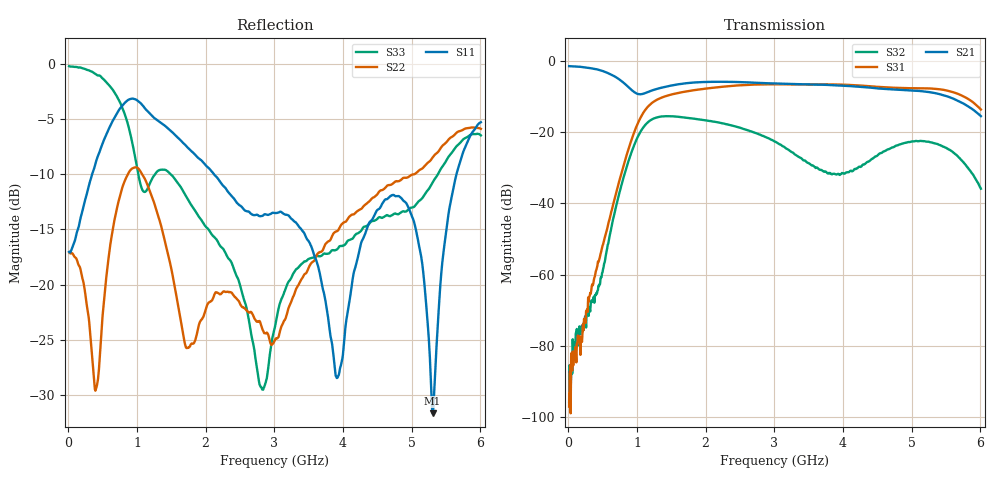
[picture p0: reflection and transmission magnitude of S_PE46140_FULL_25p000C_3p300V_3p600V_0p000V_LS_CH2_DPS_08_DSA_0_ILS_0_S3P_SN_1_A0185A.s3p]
! Device ID: PE46140_FULL
! File Path: z:\PE46140\MajorStates\25p000C\3p300\LS_CH2_DPS_08_DSA_0_ILS_0\PE46140_FULL_25p000C_3p300V_3p600V_0p000V_LS_CH2_DPS_08_DSA_0_ILS_0_S3P_SN_1_A0185A.s3p
! Serial: 1
! Lot: A0185A
! Temp: 25.000C
! VDD: 3.300
! VSS: 0.000
! Control_Hi: 3.600
! Control_Lo: 0.000
! Logic State: LS_CH2_DPS_08_DSA_0_ILS_0
! Port 1: RFIN
! Port 2: RFOUT1
! Port 3: RFOUT2
! ThroughPath:1-3
! IDD: 0.0003147101
! ISS: -1.246e-007
! Comment:
#  Hz  S  RI  R  50
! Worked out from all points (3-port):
!   801 points, 10 MHz to 6.01 GHz, reference 50 ohm
!   strongest paths, dB at 10 MHz, 1.51 GHz, 3.01 GHz, 4.51 GHz, 6.01 GHz:
!     S21: -1.5, -6.9, -6.4, -7.7, -15.5
!     S31: -97.0, -9.4, -6.6, -7.3, -13.7
!     S32: -95.7, -15.6, -22.7, -26.4, -35.9
!   lowest |S11| = -31.6 dB at 5.305 GHz (marker M1), VSWR 1.05, Z = 51.5 + j2.17 ohm
!   |S11| at or under -10 dB: start of sweep to 346.1 MHz; 2.119 GHz to 5.655 GHz (3.536 GHz wide, 91 % of centre)
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1e7  0.1402 -0.0109  0.842 -0.0245  -3.11e-05 3.34e-05
     0.8419 -0.0242  0.14 -0.00675  1.58e-05 1.55e-05
     -1.01e-05 -9.83e-06  1.38e-05 -8.72e-06  0.9729 -0.0266
4.075e8  -0.0696 -0.3583  0.3635 -0.6663  0.000303 -0.00112
         0.3648 -0.6704  -0.0311 -0.0145  -0.000562 3.68e-05
         0.000331 -0.00113  -0.000553 6.15e-05  0.5169 -0.7258
7.375e8  -0.5113 -0.3462  -0.1878 -0.5186  -0.00166 -0.02
         -0.1874 -0.5191  0.1397 0.1984  -0.0126 -0.00431
         -0.00172 -0.02  -0.0127 -0.00436  -0.1877 -0.6549
1.1425e9  -0.5829 0.1922  -0.2059 -0.2948  -0.1833 0.1181
          -0.2062 -0.2956  0.2292 -0.1731  0.0815 0.1052
          -0.1841 0.1181  0.0814 0.1053  -0.1694 -0.2075
1.8475e9  -0.1906 0.3363  -0.4832 0.1206  0.3783 -0.0913
          -0.4835 0.1205  0.0506 -0.0238  -0.15 -0.0311
          0.3789 -0.0914  -0.1503 -0.0312  -0.0922 0.1948
3.01e9  0.0105 0.2103  0.401 0.265  -0.465 -0.054
        0.4006 0.266  -0.056 -0.00182  0.0464 -0.0566
        -0.4655 -0.0545  0.0465 -0.0568  0.0203 0.0612
4.0675e9  -0.0237 -0.071  0.0104 -0.4443  0.1863 0.4218
          0.0112 -0.4445  0.1477 0.1313  0.0273 0.000723
          0.1865 0.4214  0.0273 0.000556  0.1366 0.0787
4.8475e9  -0.2447 0.0306  -0.3903 0.0197  0.3973 -0.1199
          -0.3909 0.0191  0.2977 0.0176  -0.0627 0.0265
          0.3976 -0.1199  -0.0625 0.0267  0.2115 -0.0201
5.305e9  0.0155 0.0211  -0.1485 0.3258  0.1531 -0.3784
         -0.1494 0.3259  0.3739 -0.0337  0.0347 0.0621
         0.1533 -0.3781  0.0347 0.062  0.2892 -0.0122
6.01e9  -0.361 -0.4054  0.1617 0.042  -0.187 -0.0894
        0.1622 0.0423  0.2477 -0.4421  0.00467 -0.0155
        -0.1877 -0.0887  0.00445 -0.0154  0.2914 -0.3729
